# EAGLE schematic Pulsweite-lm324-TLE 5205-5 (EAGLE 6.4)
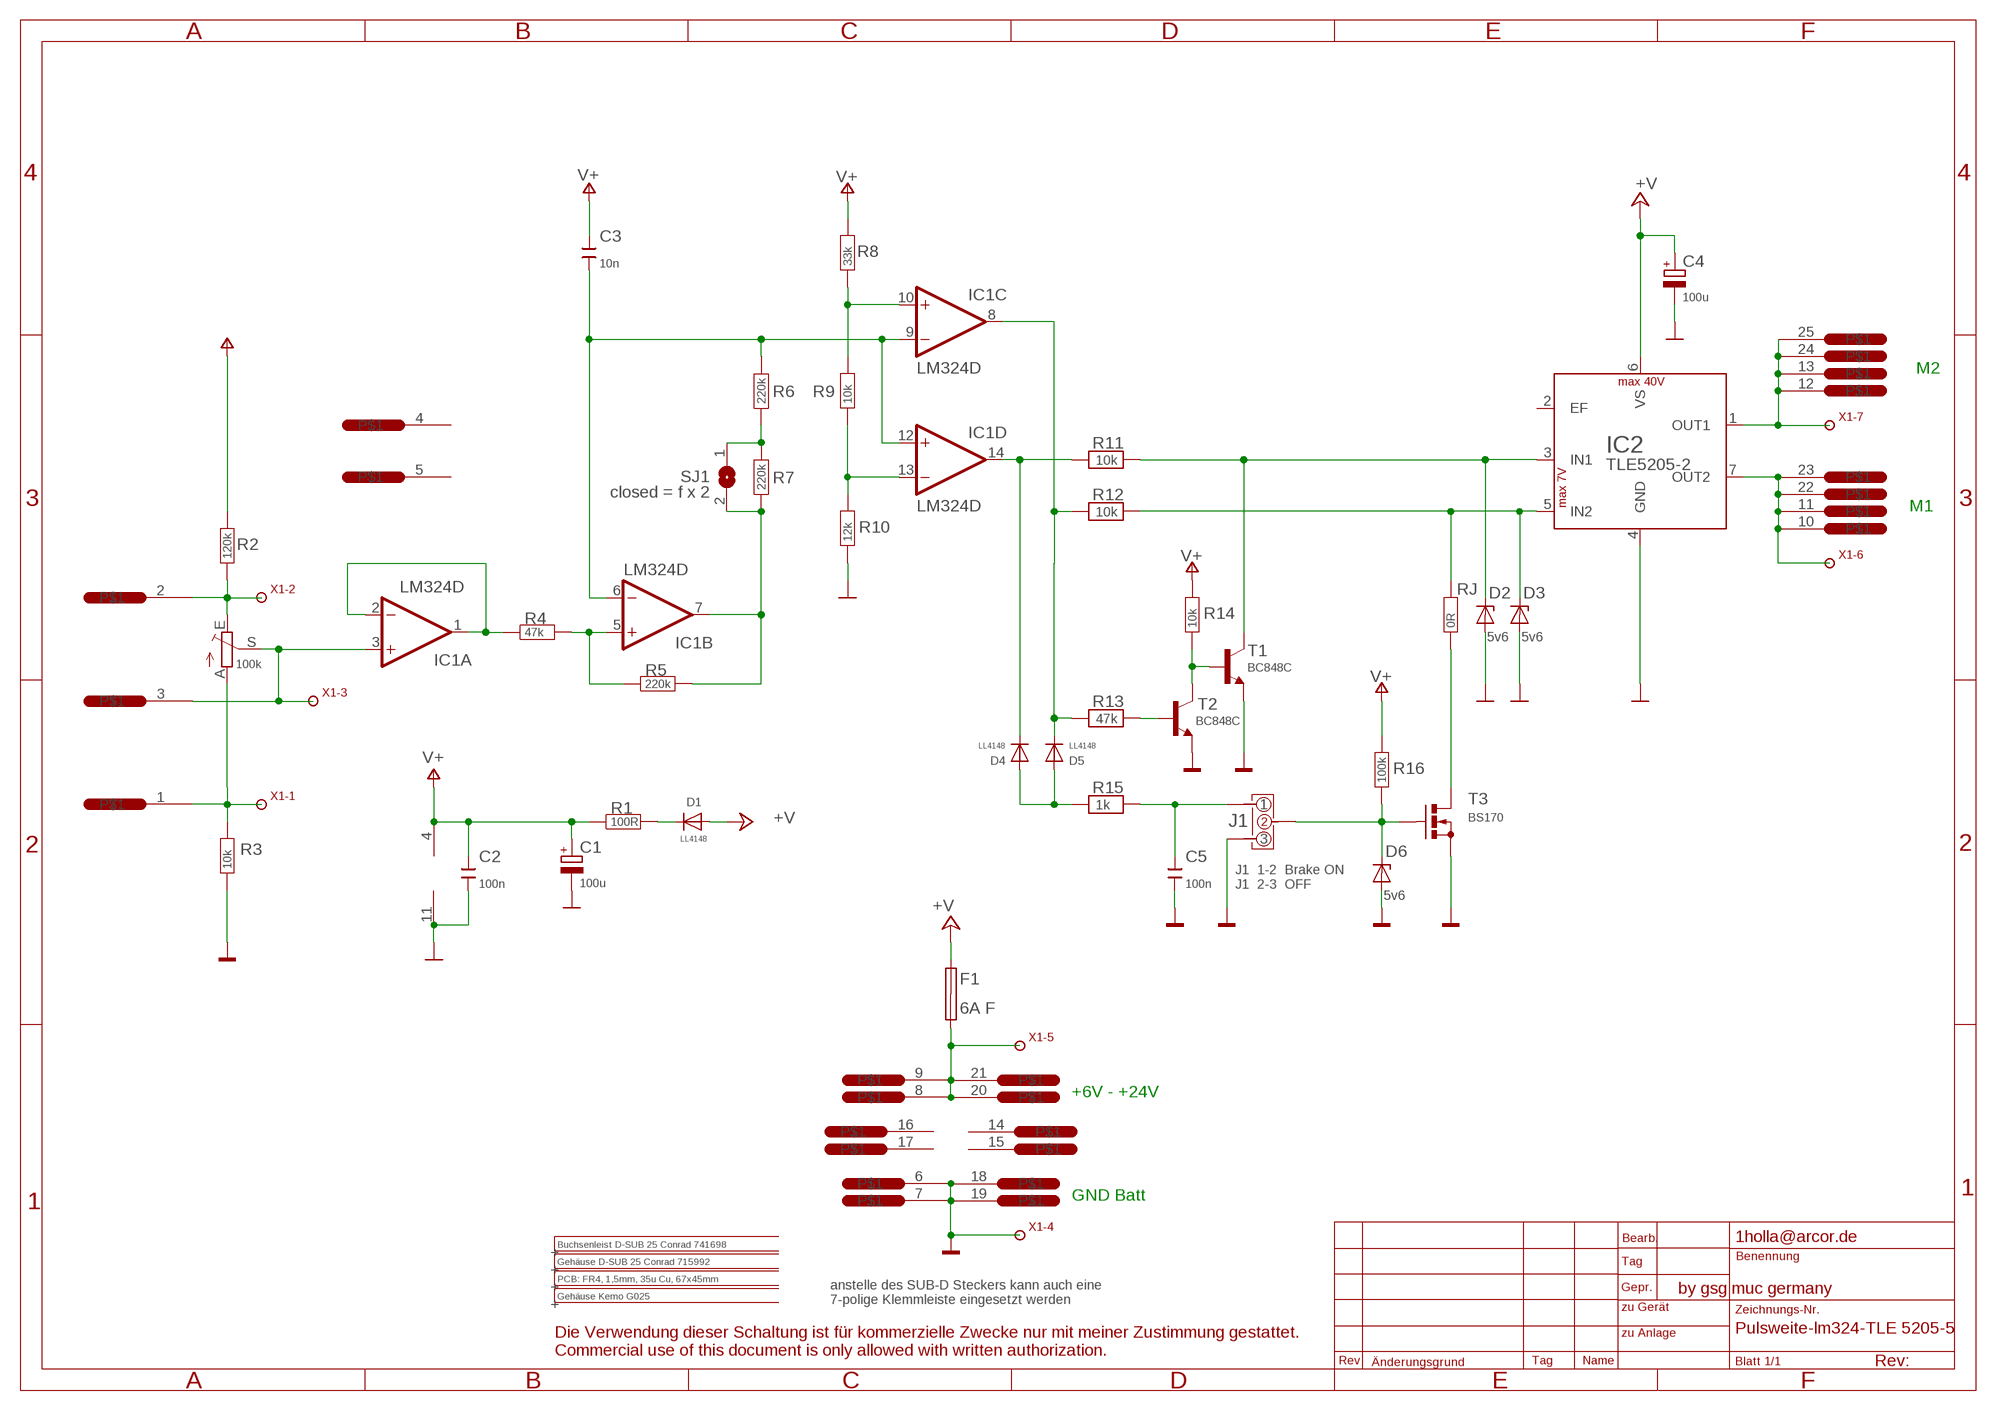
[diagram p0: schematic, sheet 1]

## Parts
..1  PCB: FR4, 1,5mm, 35u Cu, 67x45mm  INFO  [INFO]
..2  Gehäuse D-SUB 25 Conrad 715992  INFO  [INFO]
..3  Buchsenleist D-SUB 25 Conrad 741698  INFO  [INFO]
C1  100u  CPOL-EU153CLV-0810  [153CLV-0810]
C2  100n  C-EUC1206  [C1206]
C3  10n  C-EUC1206  [C1206]
C4  100u  CPOL-EU153CLV-0810  [153CLV-0810]
C5  100n  C-EUC1206  [C1206]
D1  LL4148  LL4148MELF-LM34  [MELF-LM34]
D2  5v6  ZENER-DIODESOD80C  [SOD80C]
D3  5v6  ZENER-DIODESOD80C  [SOD80C]
D4  LL4148  LL4148MELF-LM34  [MELF-LM34]
D5  LL4148  LL4148MELF-LM34  [MELF-LM34]
D6  5v6  ZENER-DIODESOD80C  [SOD80C]
ENCLOSURE-1  Gehäuse Kemo G025  KEMO-G02_  [KEMO-G02_]
F1  6A F  SHK20L  [SHK20L]
IC1  LM324D  [SO14]
IC2  TLE5205-2  [TO220-7]
J1  JP-3-THD  [JP-3]
P1  100k  TRIM_EU-LI15  [LI15]
R1  100R  R-EU_1206_S  [1206-S]
R2  120k  R-EU_1206_S  [1206-S]
R3  10k  R-EU_1206_S  [1206-S]
R4  47k  R-EU_1206_S  [1206-S]
R5  220k  R-EU_1206_S  [1206-S]
R6  220k  R-EU_1206_S  [1206-S]
R7  220k  R-EU_1206_S  [1206-S]
R8  33k  R-EU_1206_S  [1206-S]
R9  10k  R-EU_1206_S  [1206-S]
R10  12k  R-EU_1206_S  [1206-S]
R11  10k  R  [1206]
R12  10k  R  [1206]
R13  47k  R  [1206]
R14  10k  R-EU_1206_S  [1206-S]
R15  1k  R  [1206]
R16  100k  R-EU_1206_S  [1206-S]
RJ  0R  R-EU_1206_S  [1206-S]
SJ1  closed = f x 2  SJ  [SJ]
ST  D-SUB25 Conrad 741671  SUBD25LP25POL  [SUBD25LP]
T1  BC848C  BC848CLT1SMD  [SOT23]
T2  BC848C  BC848CLT1SMD  [SOT23]
T3  BS170  BS170SOT23  [SOT23]
X1  KL7  [CLAMP-07]

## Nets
6-24V: C4.+ D1.2 F1.1A IC2.6(VS) ; supply symbol labelled +V
GND: C1.- C2.2 C4.- C5.2 D2.A D3.A D6.A IC1.11(P:V-) IC2.4(GND) J1.3 R3.1 R10.1 ST.6 ST.7 ST.18 ST.19 T1.2(E) T2.2(E) T3.2(S) X1.4
M1: IC2.7(OUT2) ST.10 ST.11 ST.22 ST.23 X1.6
M2: IC2.1(OUT1) ST.12 ST.13 ST.24 ST.25 X1.7
N$1: P1.A R3.2 ST.1 X1.1
N$2: P1.E R2.1 ST.2 X1.2
N$3: IC1.3(A:+IN) P1.S ST.3 X1.3
N$4: IC1.1(A:OUT) IC1.2(A:-IN) R4.1
N$5: IC1.5(B:+IN) R4.2 R5.1
N$6: IC1.7(B:OUT) R5.2 R7.1 SJ1.2
N$7: D1.1 R1.2
N$8: C3.2 IC1.6(B:-IN) IC1.9(C:-IN) IC1.12(D:+IN) R6.2
N$9: IC1.10(C:+IN) R8.1 R9.2
N$10: IC1.13(D:-IN) R9.1 R10.2
N$11: C5.1 J1.1 R15.1
N$13: D3.C IC2.5(IN2) R12.1 RJ.2
N$14: D2.C IC2.3(IN1) R11.1 T1.3(C)
N$15: D5.1 IC1.8(C:OUT) R12.2 R13.2
N$16: F1.2A ST.8 ST.9 ST.20 ST.21 X1.5
N$17: D4.1 IC1.14(D:OUT) R11.2
N$19: R13.1 T2.1(B)
N$20: R14.1 T1.1(B) T2.3(C)
N$21: RJ.1 T3.3(D)
N$22: R6.1 R7.2 SJ1.1
N$24: D4.2 D5.2 R15.2
N$25: D6.C J1.2 R16.1 T3.1(G)
V+: C1.+ C2.1 C3.1 IC1.4(P:V+) R1.1 R2.2 R8.2 R14.2 R16.2
Unconnected: F1.1B F1.2B IC2.2(EF) ST.4 ST.5 ST.14 ST.15 ST.16 ST.17

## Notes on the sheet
- M2
- M1
- J1  1-2  Brake ON
  J1  2-3  OFF
- +6V - +24V
- GND Batt
- 1holla@arcor.de
- by gsg muc germany
- anstelle des SUB-D Steckers kann auch eine 
  7-polige Klemmleiste eingesetzt werden
- Die Verwendung dieser Schaltung ist für kommerzielle Zwecke nur mit meiner Zustimmung gestattet.
  Commercial use of this document is only allowed with written authorization.

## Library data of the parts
..1-..3 = frames:INFO
C1 C4 = rcl:CPOL-EU: POLARIZED CAPACITOR, European symbol
C2 C3 C5 = rcl:C-EU: CAPACITOR, European symbol
D1 D4 D5 = ALLGEM:LL4148
D2 D3 D6 = diode:ZENER-DIODE: Z-Diode
ENCLOSURE-1 = Enclosures-DIN-Rail+more:KEMO-G02_; ENCLOSURES: ENCLOSURE-KEMO-G020,G024,G025,G026,G028
F1 = fuse:SHK20L: FUSE HOLDER 5 x 20 mm, SH contact, SHH1 Schukat, E1073 Buerklin
IC1 = linear:LM324: OP AMP
IC2 = ALLGEM:TLE5205-2
J1 = sastec:JP-3
P1 = pot:TRIM_EU-: POTENTIOMETER
R1-R10 R14 R16 RJ = rcl:R-EU_: RESISTOR, European symbol
R11-R13 R15 = condev:R
SJ1 = jumper:SJ: SMD solder JUMPER
ST = sastec:SUBD25LP
T1 T2 = transistor-npn:BC848*: NPN Transistor
T3 = transistor-small-signal:BS170: N-CHANNEL MOS FET
X1 = CONNECT:KL7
